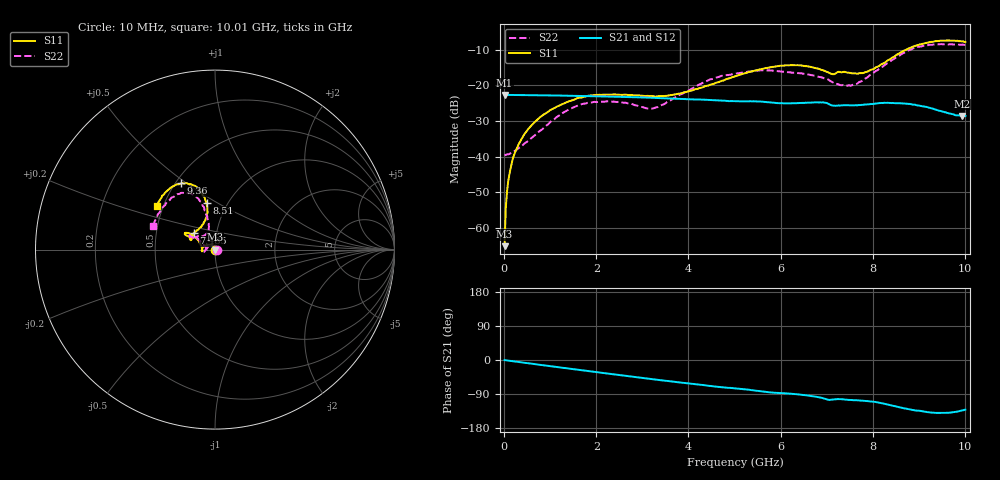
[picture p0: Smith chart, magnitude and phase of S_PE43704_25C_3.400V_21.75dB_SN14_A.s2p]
! Device ID: PE43704
! Dir: z:\PE43704\PE43704_Char_1_20130516\PE43704\AMB\3p400V\21p75dB
! Serial: 14
! Insertion: A
! Impedance: 50 ohm
! Temp: Amb
! VDD: 3.400V
! Attenuation Step: 21.75dB
! IDD: 1.139414e-01mA
#  Hz  S  RI  R  50
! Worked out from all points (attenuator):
!   401 points, 10 MHz to 10.01 GHz, reference 50 ohm
!   highest |S21| = -22.72 dB at 10 MHz (marker M1); lowest = -28.7 dB at 9.935 GHz (marker M2)
!   lowest |S11| = -65.1 dB at 10 MHz (marker M3), VSWR 1.00, Z = 50 + j0.0434 ohm
!   |S11| at or under -10 dB: start of sweep to 8.73 GHz
!   |S22| runs from -39.7 to -8.5 dB; largest |S21 - S12| = 0.00068
!   S11 on the Smith chart (normalised r, x): 10 MHz: 1.00, +0.00; 7.485 GHz: 0.78, +0.15; 8.51 GHz: 0.80, +0.45; 9.36 GHz: 0.53, +0.48; 10.01 GHz: 0.46, +0.27
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1e7  0.000343 0.000434  0.0731 -0.000228  0.0731 -0.000238  0.0103 0.000324
8.5e7  0.00046 0.00432  0.073 -0.0019  0.073 -0.00187  0.0103 0.00308
1.35e8  0.00024 0.0066  0.0729 -0.00296  0.0729 -0.00294  0.0099 0.00497
2.35e8  -0.00137 0.0113  0.0726 -0.00504  0.0727 -0.00499  0.00824 0.00876
3.85e8  -0.00453 0.0173  0.0723 -0.00826  0.0721 -0.00815  0.00478 0.0132
8.35e8  -0.0246 0.0288  0.0701 -0.017  0.0701 -0.0169  -0.0144 0.0196
1.685e9  -0.0657 0.0146  0.0629 -0.0321  0.0629 -0.0321  -0.0543 -0.00114
2.26e9  -0.0737 -0.00271  0.0561 -0.0407  0.0561 -0.0406  -0.0572 -0.0152
3.36e9  -0.0705 -0.00156  0.0399 -0.0525  0.0399 -0.0525  -0.0492 0.00833
4.41e9  -0.0884 0.0425  0.0238 -0.0577  0.0239 -0.0577  -0.0968 0.0625
5.01e9  -0.1125 0.071  0.0156 -0.0577  0.0157 -0.0576  -0.126 0.0709
5.96e9  -0.1602 0.094  0.003 -0.0559  0.00317 -0.056  -0.1402 0.0694
6.685e9  -0.1606 0.0796  -0.00534 -0.0569  -0.00558 -0.0568  -0.1216 0.0652
7.11e9  -0.1302 0.0613  -0.013 -0.0504  -0.0132 -0.0505  -0.0829 0.0754
7.485e9  -0.1169 0.0936  -0.0138 -0.0503  -0.014 -0.0505  -0.0512 0.0856
7.835e9  -0.0739 0.1336  -0.0166 -0.0509  -0.0166 -0.0509  -0.0351 0.1188
8.36e9  -0.0424 0.2246  -0.0271 -0.0495  -0.027 -0.0498  -0.0503 0.2056
8.51e9  -0.0455 0.2596  -0.0304 -0.0469  -0.0302 -0.047  -0.0627 0.238
8.935e9  -0.0973 0.3444  -0.0362 -0.0384  -0.0361 -0.0382  -0.1297 0.3091
9.36e9  -0.188 0.3699  -0.0348 -0.0295  -0.0348 -0.0297  -0.2183 0.305
9.935e9  -0.3121 0.2693  -0.0253 -0.0269  -0.0258 -0.027  -0.3346 0.1599
1.001e10  -0.324 0.2431  -0.0242 -0.028  -0.0249 -0.028  -0.3442 0.1304
